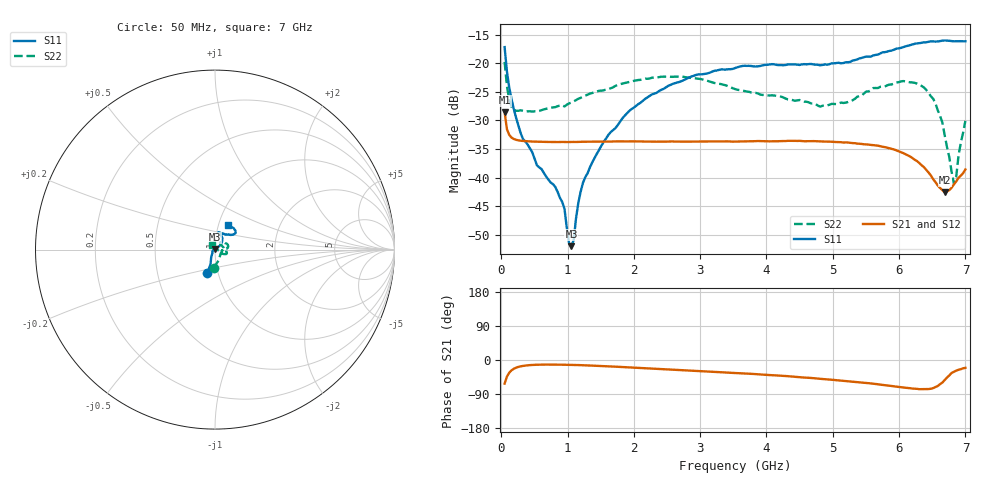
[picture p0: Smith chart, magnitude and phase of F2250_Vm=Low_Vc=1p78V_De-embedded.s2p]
! Integrated Device Technology
! Corporate Headquarters
! 6024 Silver Creek Valley Road
! San Jose, CA 95138  USA
! Phone:  1-408-284-8200
! Toll Free:  1-800-223-1366
! Webpage:  http://www.idt.com/
! Timing and RF Division
! 515 Groton Road, Suite 102
! Westford, MA 01886-6024
! Device:  F2250
! Description: Voltage Variable RF Attenuator
! Frequency:  50.0 -  6000.00 MHz
! Package:  3x3 mm Thin QFN Plastic Package: 16 pin
! Ports:  2 RF, 3 DC
!  Pin  1  = GND
!  Pin  2  = NC
!  Pin  3  = RF1  = Port 1
!  Pin  4  = NC
!  Pin  5  = GND
!  Pin  6  = GND
!  Pin  7  = GND
!  Pin  8  = GND
!  Pin  9  = NC
!  Pin 10  = RF2  = Port 2
!  Pin 11  = NC
!  Pin 12  = GND
!  Pin 13  = GND
!  Pin 14  = VCNTRL
!  Pin 15  = VDD
!  Pin 16  = VMODE
! Vcntrl:  1.780 Volts
! Vmode:  +0.000 Volts
! Vdd:  +3.30  Volts
! Current:  1.187 mA
! Data:  The device was measured on a the F2250 evaluation board which has
!  individual transmission lines to the RF pins.  Data was collected
!  using a calibrated network analyzer.  The evaluation board was
!  de-embedded using a TRL calibration technique.
!  The reference plane is the edge of the package pin.
! Misc:  SN 10
!  Action Tracker AT0258
! Date Measured:  2014-11-26
! Date:  2015-10-15  MJV
! Note:
!  Integrated Device Technology supplies this data as a sample of measured
!  data at the package pin for this product.  Your particular data for this
!  product may vary.
!  Data was taken at 25 degrees C.
!  Integrated Device Technology reserves the right to change this data at anytime.
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# GHz S dB R 50
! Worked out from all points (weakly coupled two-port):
!   201 points, 50 MHz to 7 GHz, reference 50 ohm
!   highest |S21| = -28.57 dB at 50 MHz (marker M1); lowest = -42.6 dB at 6.687 GHz (marker M2)
!   lowest |S11| = -52.0 dB at 1.058 GHz (marker M3), VSWR 1.01, Z = 49.9 + j0.227 ohm
!   |S11| at or under -10 dB: start of sweep to end of sweep
!   |S22| runs from -41.0 to -19.8 dB; largest |S21 - S12| = 4.9e-05
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0.05  -17.17 -108.3  -28.57 -62.2  -28.56 -62.2  -19.76 -94.6
0.1195  -24.20 -111.2  -32.53 -33.5  -32.54 -33.5  -26.37 -57.1
0.189  -28.02 -118.9  -33.25 -23.1  -33.24 -23.1  -28.10 -38.7
0.328  -33.27 -132.6  -33.60 -15.5  -33.60 -15.5  -28.32 -19.3
0.91875  -44.27 157.7  -33.76 -12.4  -33.77 -12.4  -27.34 -5.3
0.9535  -45.49 170.2  -33.78 -12.5  -33.78 -12.5  -27.56 -4.1
1.023  -51.57 141.8  -33.77 -12.7  -33.78 -12.7  -27.01 -2.4
1.05775  -52.00 115.2  -33.77 -12.9  -33.77 -12.9  -26.86 -1.8
1.2315  -40.93 40.9  -33.73 -13.8  -33.73 -13.8  -25.86 -2.8
1.6485  -32.06 40.7  -33.70 -17.0  -33.69 -17.0  -24.38 3.8
2.37825  -24.87 46.8  -33.71 -23.5  -33.71 -23.5  -22.43 13.7
3.525  -20.83 72.3  -33.70 -34.2  -33.71 -34.2  -24.51 39.2
4.7065  -20.21 72.2  -33.62 -48.0  -33.62 -48.0  -27.03 47.0
5.193  -19.82 57.0  -33.85 -55.3  -33.85 -55.3  -26.90 22.4
5.85325  -17.84 40.3  -34.88 -67.8  -34.88 -67.9  -23.73 -10.1
6.3745  -16.35 41.3  -38.17 -77.0  -38.18 -77.0  -24.24 -24.2
6.54825  -16.21 45.0  -40.79 -71.5  -40.79 -71.5  -27.01 -27.9
6.68725  -16.01 48.7  -42.60 -52.9  -42.57 -52.8  -32.56 -17.2
6.82625  -16.15 53.5  -41.19 -31.2  -41.15 -31.1  -41.03 49.0
6.861  -16.14 55.0  -40.69 -28.1  -40.66 -28.1  -39.95 73.6
6.89575  -16.11 57.0  -40.05 -25.9  -40.04 -25.8  -36.19 92.5
7  -16.14 63.1  -38.58 -20.7  -38.56 -20.7  -30.07 118.0
